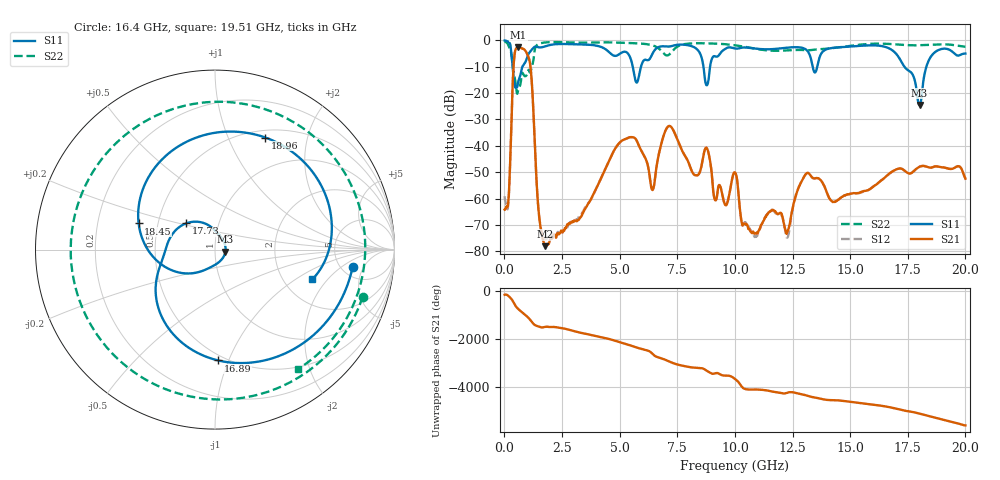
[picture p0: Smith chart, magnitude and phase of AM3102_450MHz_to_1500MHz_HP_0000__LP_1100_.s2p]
!Agilent Technologies,E8364B,MY43040894,A.07.50.67
!Agilent E8364B: A.07.50.67
!Date: Thursday, January 11, 2018 05:18:10
!Correction: S11(Full 2 Port(1,2))
!S21(Full 2 Port(1,2))
!S12(Full 2 Port(1,2))
!S22(Full 2 Port(1,2))
!S2P File: Measurements: S11, S21, S12, S22:
# Hz S  dB  R 50
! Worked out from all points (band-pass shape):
!   1601 points, 10 MHz to 20 GHz, reference 50 ohm
!   highest |S21| = -2.68 dB at 609.7 MHz (marker M1); lowest = -78.1 dB at 1.772 GHz (marker M2)
!   |S21| within 3 dB of the highest: 437.4 MHz to 1.014 GHz (576.1 MHz wide, 79.4 % of centre)
!   lowest |S11| = -24.6 dB at 18.01 GHz (marker M3), VSWR 1.13, Z = 56.2 - j1.28 ohm
!   |S11| at or under -10 dB: 357.6 MHz to 782.2 MHz (424.6 MHz wide, 74.5 % of centre); 5.568 GHz to 5.928 GHz (359.9 MHz wide, 6.26 % of centre); 17.35 GHz to 18.31 GHz (953.3 MHz wide, 5.35 % of centre)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
!   |S22| runs from -20.3 to -0.5 dB; largest |S21 - S12| = 0.0021
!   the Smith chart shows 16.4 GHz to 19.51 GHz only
!   S11 on the Smith chart (normalised r, x): 16.4 GHz: 6.28, -3.05; 16.89 GHz: 0.46, -0.92; 17.73 GHz: 0.70, +0.21; 18.45 GHz: 0.39, +0.14; 18.96 GHz: 0.59, +1.37; 19.51 GHz: 2.86, -1.40
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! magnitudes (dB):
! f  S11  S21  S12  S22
! 10 MHz  -0.1  -64.2  -59.1  -0.5
! 159.9 MHz  -0.5  -62.2  -62.9  -1.6
! 422.3 MHz  -15.3  -7.0  -7.0  -12.9
! 609.7 MHz  -15.4  -2.7  -2.7  -18.7
! 1.109 GHz  -4.4  -8.6  -8.6  -12.2
! 1.484 GHz  -2.6  -64.6  -64.9  -1.4
! 1.772 GHz  -2.3  -78.1  -75.3  -0.8
! 3.346 GHz  -1.6  -66.6  -66.0  -0.9
! 5.082 GHz  -4.7  -38.2  -38.2  -0.9
! 6.682 GHz  -2.6  -43.9  -44.0  -3.0
! 10.01 GHz  -3.1  -50.1  -50.1  -1.9
! 10.89 GHz  -3.1  -73.3  -74.3  -3.2
! 13.34 GHz  -8.6  -51.9  -51.9  -3.7
! 16.4 GHz  -2.2  -52.8  -52.8  -1.3
! 16.68 GHz  -3.0  -50.6  -50.8  -1.4
! 16.89 GHz  -4.2  -49.5  -49.4  -1.5
! 17.73 GHz  -13.3  -49.8  -50.0  -1.9
! 18.01 GHz  -24.6  -47.9  -47.9  -1.9
! 18.45 GHz  -6.9  -48.3  -48.3  -1.7
! 18.96 GHz  -3.3  -48.1  -48.1  -1.5
! 19.51 GHz  -4.9  -48.5  -48.4  -1.8
! 20 GHz  -5.0  -52.5  -52.4  -2.4
